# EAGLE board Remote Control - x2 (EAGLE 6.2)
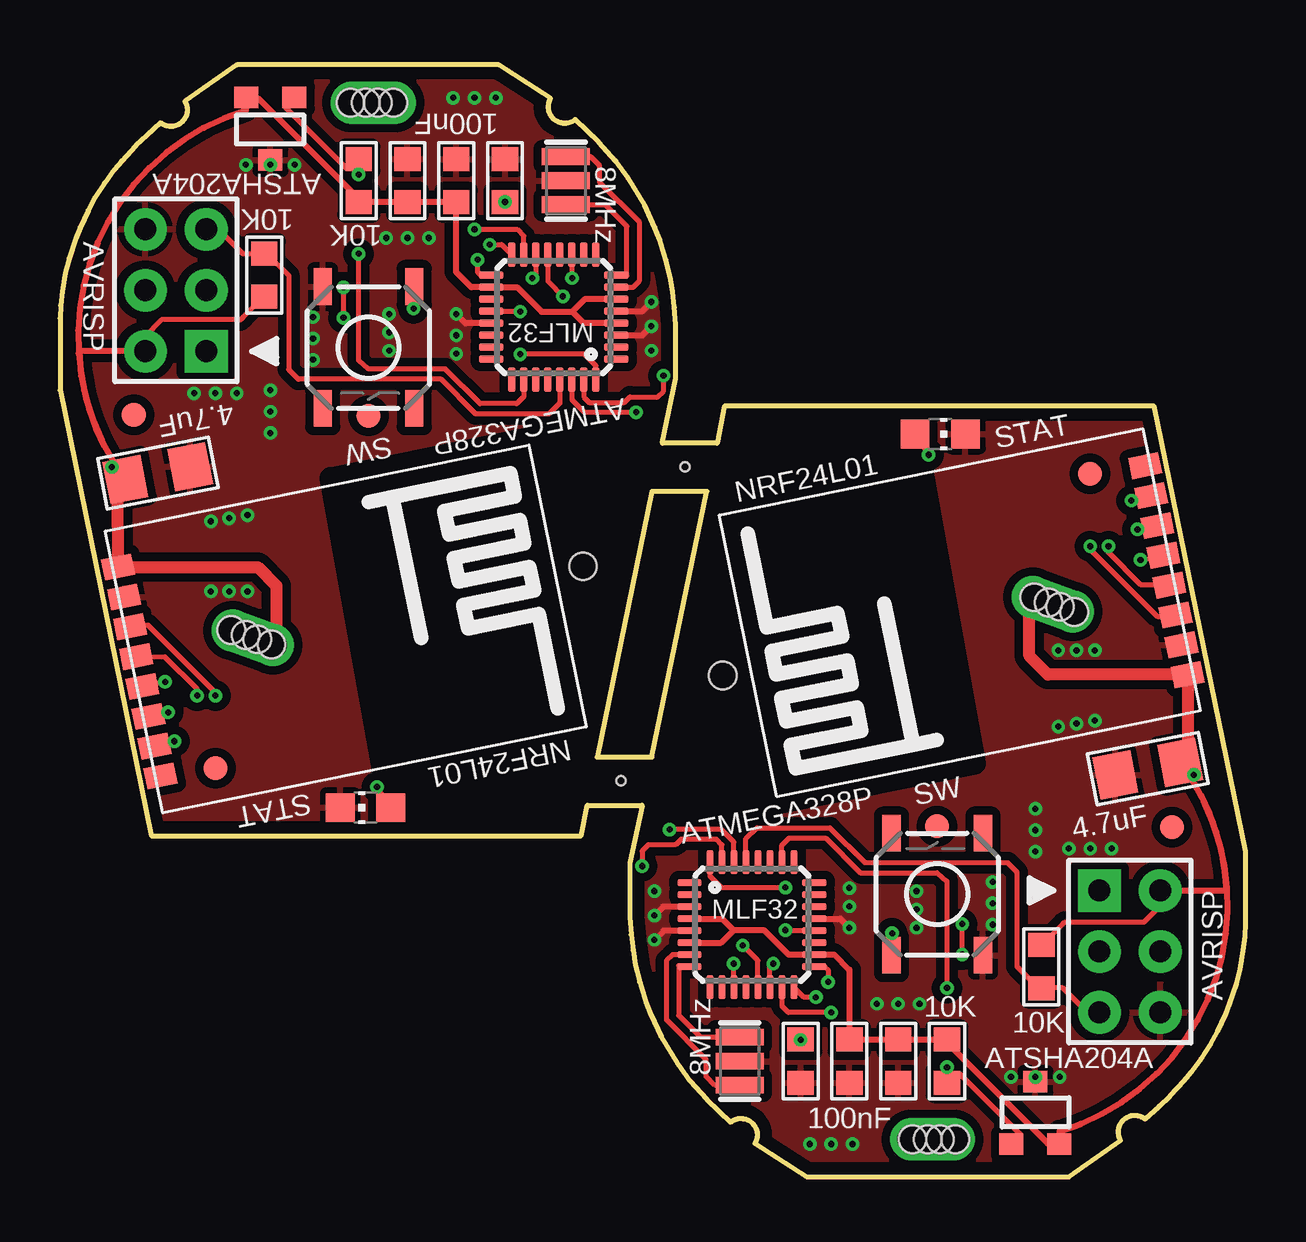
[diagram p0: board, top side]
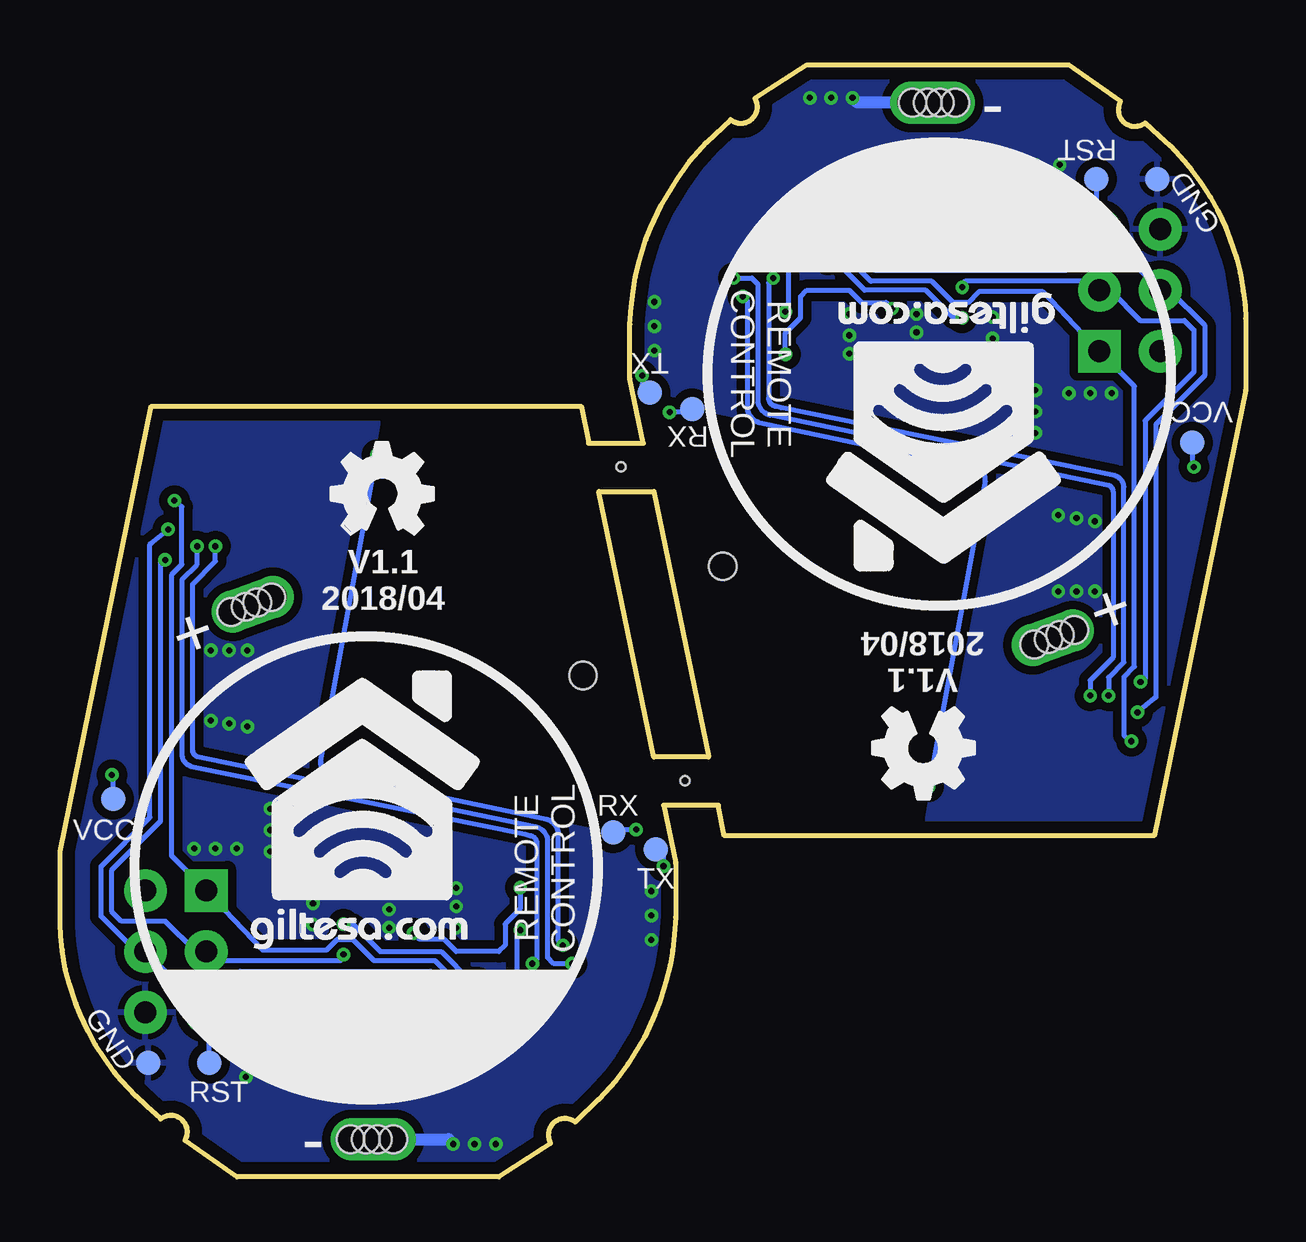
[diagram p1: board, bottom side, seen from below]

Size 49.4 x 46.35 mm. Coordinates in mm from the lower left corner, seen from the top.
Outline: 79 segments
Copper layers (1*16): Top 0.035mm / dielectric 1.6mm / Bottom 0.035mm
Design rules: minimum track width 6mil, minimum drill 12mil, track to track 6mil, track to pad 6mil, pad to pad 6mil, via to via 8mil, smd to smd 0mil, copper to edge 20mil, drill to drill 10mil, minimum pad ring 6mil, minimum via ring 6mil, stop-mask expansion 0mil, vias tented up to drill 100mil, thermal gap 10mil
Net classes: 2 gnd: width 0.305 mm, drill 0.406 mm, clearance 0.203 mm; 3 usbvcc: width 0.203 mm, drill 0.406 mm, clearance 0.203 mm; 4 USBpair: width 0.254 mm, drill 0.406 mm, clearance 0.61 mm
Holes 1.14 mm at 27.61,20.9 21.79,25.45
Holes 0.38 mm at 23.37,16.51 26.04,29.59
tRestrict: 8 lines
bRestrict: 8 lines

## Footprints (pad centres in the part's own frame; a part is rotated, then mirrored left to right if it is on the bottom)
C1206 = smd 1.6 x 1.8: 1 -1.362,0; 2 1.387,0
C0603 = smd 1 x 1.1: 1 -0.901,0; 2 0.901,0
PAD_KEYFINDER = drill 1.143 pad 1.778 offset: P$2 -0.889,0; P$3 0.889,0 | hole 1.143: -0.191,0; 0.318,0; -0.826,0; 0.953,0
HEAD3X2 = drill 0.914 pad 1.778 square: 1 0,0 | drill 0.914 pad 1.778: 2 0,2.54; 3 2.54,0; 4 2.54,2.54; 5 5.08,0; 6 5.08,2.54
CHIP-LED0805 = smd 1.2 x 1.2: A 0,-1.05; C 0,1.05
R0603 = smd 1 x 1.1: 1 -0.901,0; 2 0.901,0
SWITCH-5X5MM-SMD = smd 1.524 x 0.762: A -2.54,1.905; B -2.54,-1.905; NC@1 2.54,1.905; NC@2 2.54,-1.905
PAD.03X.04 = smd 1.016 x 1.016: P$1 0,0
SOT23-3 = smd 1 x 0.9: 1 -1,-1.3; 2 1,-1.3; 3 0,1.3
NRF24L01_SMD = smd 0.9 x 1.27: 3.3V 1.575,0.203; CE 4.115,0.203; CSN 5.385,0.203; GND 2.845,0.203; IRQ 10.465,0.203; MISO 9.195,0.203; MOSI 7.925,0.203; SCK 6.655,0.203
MLF32_HAND_SOLDERING = smd 1.016 x 0.3: 1 -2.604,1.75; 2 -2.604,1.25; 3 -2.604,0.75; 4 -2.604,0.25; 5 -2.604,-0.25; 6 -2.604,-0.75; 7 -2.604,-1.25; 8 -2.604,-1.75; 17 2.604,-1.75; 18 2.604,-1.25; 19 2.604,-0.75; 20 2.604,-0.25; 21 2.604,0.25; 22 2.604,0.75; 23 2.604,1.25; 24 2.604,1.75 | smd 0.3 x 1.016: 9 -1.75,-2.604; 10 -1.25,-2.604; 11 -0.75,-2.604; 12 -0.25,-2.604; 13 0.25,-2.604; 14 0.75,-2.604; 15 1.25,-2.604; 16 1.75,-2.604; 25 1.75,2.604; 26 1.25,2.604; 27 0.75,2.604; 28 0.25,2.604; 29 -0.25,2.604; 30 -0.75,2.604; 31 -1.25,2.604; 32 -1.75,2.604
FIDUCIAL-1X2 = smd 1 x 1: 1 0,0
RESONATOR = smd 0.7 x 2: 1 -1,0; 2 0,0; 3 1,0

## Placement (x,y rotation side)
C1  4.7uF  [C1206]  45.34,17.02 191 top
C2  4.7uF  [C1206]  4.06,29.34 11 top
C3  100nF  [C0603]  30.86,4.83 90 top
C4  100nF  [C0603]  32.89,4.83 90 top
C5  100nF  [C0603]  14.48,41.53 270 top
C6  100nF  [C0603]  18.54,41.53 270 top
C7  100nF  [C0603]  34.92,4.83 90 top
C8  100nF  [C0603]  16.51,41.53 270 top
J1  B-  [PAD_KEYFINDER]  36.35,1.57 0 top
J2  B+  [PAD_KEYFINDER]  41.37,23.88 340 top
J3  B-  [PAD_KEYFINDER]  13.06,44.78 180 top
J4  AVRISP  [HEAD3X2]  43.31,11.94 270 top
J5  B+  [PAD_KEYFINDER]  8.03,22.48 160 top
J6  AVRISP  [HEAD3X2]  6.1,34.42 90 top
L1  STAT  [CHIP-LED0805]  36.68,30.96 270 top
L2  STAT  [CHIP-LED0805]  12.73,15.39 90 top
LOGO1  OSHW_LOGO_FILLX0150-NT  [OSHW_FILLX150_NOTEXT]  38.1,26.8 0 bottom
LOGO2  OSHW_LOGO_FILLX0150-NT  [OSHW_FILLX150_NOTEXT]  11.3,19.56 180 bottom
R1  10K  [R0603]  12.45,41.53 90 top
R2  10K  [R0603]  8.51,37.59 270 top
R3  10K  [R0603]  36.96,4.83 270 top
R4  10K  [R0603]  40.89,8.76 90 top
S1  SW  [SWITCH-5X5MM-SMD]  36.55,11.79 90 top
S2  SW  [SWITCH-5X5MM-SMD]  12.85,34.57 270 top
TP1  RX  [PAD.03X.04]  26.35,14.35 0 bottom
TP2  TX  [PAD.03X.04]  24.57,13.65 0 bottom
TP3  RESET  [PAD.03X.04]  43.18,4.76 0 bottom
TP4  VCC  [PAD.03X.04]  47.18,15.75 0 bottom
TP5  GND  [PAD.03X.04]  45.72,4.76 0 bottom
TP6  RX  [PAD.03X.04]  23.05,32 180 bottom
TP7  TX  [PAD.03X.04]  24.83,32.7 180 bottom
TP8  RESET  [PAD.03X.04]  6.22,41.59 180 bottom
TP9  VCC  [PAD.03X.04]  2.22,30.61 180 bottom
TP10  GND  [PAD.03X.04]  3.68,41.59 180 bottom
U1  ATSHA204A  [SOT23-3]  8.76,43.69 180 top
U2  NRF24L01  [NRF24L01_SMD]  47.5,19.43 101.5 top
U3  ATSHA204A  [SOT23-3]  40.64,2.67 0 top
U4  NRF24L01  [NRF24L01_SMD]  1.91,26.92 281.5 top
U5  ATMEGA328P  [MLF32_HAND_SOLDERING]  28.83,10.52 0 top
U6  ATMEGA328P  [MLF32_HAND_SOLDERING]  20.57,35.84 180 top
U$1  DOMOTICA10MM  [DOMOTICA-10MM]  7.62,36.96 180 bottom
U$2  FIDUCIAL1X2  [FIDUCIAL-1X2]  12.85,31.72 180 top
U$3  FIDUCIAL1X2  [FIDUCIAL-1X2]  6.48,17.04 180 top
U$4  FIDUCIAL1X2  [FIDUCIAL-1X2]  3.07,31.78 180 top
U$5  DOMOTICA10MM  [DOMOTICA-10MM]  41.78,9.4 0 bottom
U$6  FIDUCIAL1X2  [FIDUCIAL-1X2]  36.55,14.63 0 top
U$7  FIDUCIAL1X2  [FIDUCIAL-1X2]  42.93,29.31 0 top
U$8  CC-NC-BCNIX  [CC-NC-B_NIX]  -0.38,0 180 top
U$14  FIDUCIAL1X2  [FIDUCIAL-1X2]  46.33,14.58 0 top
U$15  CC-NC-BCNIX  [CC-NC-B_NIX]  23.75,0 0 top
Y1  8MHz  [RESONATOR]  28.32,4.83 90 top
Y2  8MHz  [RESONATOR]  21.08,41.53 270 top

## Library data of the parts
C1-C8 J1-J3 J5 R1-R4 S1 S2 U2 U4-U6 = ,giltesa
J4 J6 = MyCON2
L1 L2 = led
LOGO1 LOGO2 = ohw-logo
TP1-TP10 = SparkFun-Connectors
U1 U3 = TD-MySensors
U$1 U$5 = ,giltesa_logos
U$2-U$4 U$6 U$7 U$14 = SparkFun
U$8 U$15 = cc-by-nc-sa
Y1 Y2 = MySMD2

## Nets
A3_ATSHA204A: R3.2 U3.1 U5.26
A3_ATSHA204A1: R1.2 U1.1 U6.26
D2_INT_SW: S1.A U5.32
D2_INT_SW1: S2.A U6.32
D7_RF_CE: U2.CE U5.11
D7_RF_CE1: U4.CE U6.11
D9_LEDB~: L1.A U5.13
D9_LEDB~1: L2.A U6.13
D10_RF_CS: U2.CSN U5.14
D10_RF_CS1: U4.CSN U6.14
D11_MOSI: J4.4 U2.MOSI U5.15
D11_MOSI1: J6.4 U4.MOSI U6.15
D12_MISO: J4.1 U2.MISO U5.16
D12_MISO1: J6.1 U4.MISO U6.16
D13_SCK: J4.3 U2.SCK U5.17
D13_SCK1: J6.3 U4.SCK U6.17
GND [gnd]: C1.2 C3.1 C4.1 C7.1 J1.P$2 J4.6 L1.C S1.B TP5.P$1 U2.GND U3.3 U5.3 U5.5 U5.21 Y1.2
GND1 [gnd]: C2.2 C5.1 C6.1 C8.1 J3.P$2 J6.6 L2.C S2.B TP10.P$1 U1.3 U4.GND U6.3 U6.5 U6.21 Y2.2
N$1: TP1.P$1 U5.30
N$2: TP2.P$1 U5.31
N$3: C6.2 U6.20
N$4: TP6.P$1 U6.30
N$5: TP7.P$1 U6.31
N$6: U6.7 Y2.1
N$7: U6.8 Y2.3
N$29: U5.7 Y1.1
N$30: U5.8 Y1.3
N$33: C3.2 U5.20
RESET: J4.5 R4.1 TP3.P$1 U5.29
RESET1: J6.5 R2.1 TP8.P$1 U6.29
VCC: C1.1 C4.2 C7.2 J2.P$2 J4.2 R3.1 R4.2 TP4.P$1 U2.3.3V U3.2 U5.4 U5.6 U5.18
VCC1: C2.1 C5.2 C8.2 J5.P$2 J6.2 R1.1 R2.2 TP9.P$1 U1.2 U4.3.3V U6.4 U6.6 U6.18

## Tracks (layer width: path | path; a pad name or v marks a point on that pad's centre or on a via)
A3_ATSHA204A  (via drill 0.25)
  Top 0.203: U5.26 30.08,13.82 30.38,14.12 31.9,14.12 33.35,12.68 36.55,12.68 36.96,12.32 v36.96,7.87 | U3.1 40.01,1.73 40.01,1.78 37.46,4.32 37.08,4.32 v36.96,4.57 R3.2
  Bottom 0.203: v36.96,7.87 v36.96,4.57
A3_ATSHA204A1  (via drill 0.25)
  Top 0.203: U6.26 19.32,32.53 19.02,32.23 17.5,32.23 16.05,33.68 12.85,33.68 12.45,34.04 v12.45,38.48 | U1.1 9.4,44.62 9.4,44.58 11.94,42.04 12.32,42.04 v12.45,41.78 R1.2
  Bottom 0.203: v12.45,38.48 v12.45,41.78
D2_INT_SW  (via drill 0.25)
  Top 0.203: U5.32 27.08,12.54 27.56,12.06 v30.23,12.06 | S1.A 34.65,10.13 v34.67,10.16
  Bottom 0.203: v34.67,10.16 34.42,9.91 33.4,9.91 32.89,9.4 31.11,9.4 30.86,9.65 30.86,10.54 30.23,11.18 v30.23,12.06
D2_INT_SW1  (via drill 0.25)
  Top 0.203: U6.32 22.32,33.81 21.84,34.29 v19.18,34.29 | S2.A 14.76,36.22 v14.73,36.2
  Bottom 0.203: v14.73,36.2 14.99,36.45 16,36.45 16.51,36.96 18.29,36.96 18.54,36.7 18.54,35.81 19.18,35.18 v19.18,34.29
D7_RF_CE  (via drill 0.25)
  Top 0.203: U5.11 28.08,8.88 v28.07,8.89 | v42.93,26.29 42.93,26.16 45.72,23.37 46.45,23.37 U2.CE
  Bottom 0.203: v28.07,8.89 28.83,8.89 29.08,9.14 29.08,14.03 arc-70 29.59,14.61 43.69,17.53 arc70 43.88,17.78 43.88,24.7 42.93,25.65 v42.93,26.29
D7_RF_CE1  (via drill 0.25)
  Top 0.203: U6.11 21.32,37.48 v21.34,37.47 | v6.48,20.07 6.48,20.19 3.68,22.99 2.95,22.99 U4.CE
  Bottom 0.203: v21.34,37.47 20.57,37.47 20.32,37.21 20.32,32.32 arc-70 19.81,31.75 5.71,28.83 arc70 5.52,28.57 5.52,21.65 6.48,20.7 v6.48,20.07
D9_LEDB~  (via drill 0.25)
  Top 0.203: v36.2,30.1 L1.A | U5.13 29.08,9.02 v28.45,9.65
  Bottom 0.203: v36.2,30.1 38.54,17.34 arc-90 38.16,16.83 29.15,14.92 arc70 28.64,14.29 28.64,9.84 v28.45,9.65
D9_LEDB~1  (via drill 0.25)
  Top 0.203: v13.21,16.26 L2.A | U6.13 20.32,37.33 v20.95,36.7
  Bottom 0.203: v13.21,16.26 10.86,29.02 arc-90 11.24,29.53 20.26,31.43 arc70 20.76,32.07 20.76,36.51 v20.95,36.7
D10_RF_CS  (via drill 0.25)
  Top 0.203: 46.06,24.89 46.06,24.72 | 46.06,24.72 45.85,24.51 | U5.14 29.58,8.75 v29.72,8.89 | v43.69,26.29 43.69,26.02 45.03,24.68 U2.CSN 46.23,24.72 46.06,24.72
  Bottom 0.203: v29.72,8.89 29.53,9.08 29.53,13.91 arc-70 29.78,14.22 30.04,14.29 43.94,17.12 arc70 44.32,17.59 44.32,24.89 43.69,25.53 v43.69,26.29
D10_RF_CS1  (via drill 0.25)
  Top 0.203: 3.35,21.46 3.35,21.63 | 3.35,21.63 3.56,21.84 | U6.14 19.82,37.6 v19.68,37.47 | v5.71,20.07 5.71,20.33 4.37,21.68 U4.CSN 3.17,21.63 3.35,21.63
  Bottom 0.203: v19.68,37.47 19.88,37.27 19.88,32.45 arc-70 19.62,32.13 19.37,32.07 5.46,29.23 arc70 5.08,28.77 5.08,21.46 5.71,20.83 v5.71,20.07
D11_MOSI  (via drill 0.25)
  Top 0.203: 45.85,27.18 45.85,27.11 U2.MOSI v44.9,26.99 | v32.13,6.86 30.35,6.86 30.08,7.13 U5.15
  Bottom 0.203: v44.9,26.99 45.59,26.42 45.66,26.35 45.66,14.99 47.69,12.95 47.69,10.86 46.23,9.4 J4.4 44.58,8.13 42.35,8.13 41.91,8.57 33.97,8.57 32.26,6.86 v32.13,6.86
D11_MOSI1  (via drill 0.25)
  Top 0.203: 3.56,19.18 3.56,19.24 U4.MOSI v4.51,19.37 | v17.27,39.5 19.05,39.5 19.32,39.22 U6.15
  Bottom 0.203: v4.51,19.37 3.81,19.94 3.75,20 3.75,31.37 1.71,33.4 1.71,35.5 3.17,36.96 J6.4 4.83,38.23 7.05,38.23 7.49,37.78 15.43,37.78 17.14,39.5 v17.27,39.5
D12_MISO  (via drill 0.25)
  Top 0.203: v44.64,28.19 U2.MISO | v31.5,7.49 31,7.49 U5.16
  Bottom 0.203: v44.64,28.19 44.32,27.94 44.32,25.53 44.77,25.08 44.77,13.4 J4.1 42.93,11.56 40.96,9.46 38.29,9.46 37.85,9.91 37.21,9.91 36.32,9.02 33.78,9.02 32.26,7.49 v31.5,7.49
D12_MISO1  (via drill 0.25)
  Top 0.203: v4.76,18.16 U4.MISO | v17.91,38.86 18.41,38.86 U6.16
  Bottom 0.203: v4.76,18.16 5.08,18.41 5.08,20.83 4.63,21.27 4.63,32.96 J6.1 6.48,34.8 8.45,36.89 11.11,36.89 11.56,36.45 12.19,36.45 13.08,37.34 15.62,37.34 17.14,38.86 v17.91,38.86
D13_SCK  (via drill 0.25)
  Top 0.203: v45.02,25.72 U2.SCK | v37.59,9.27 v37.59,10.54 | U5.17 31.87,8.77 32,8.64 v32,8.13
  Bottom 0.203: v45.02,25.72 45.21,25.59 45.21,14.83 47.24,12.8 47.24,11.05 46.85,10.65 45.01,10.65 43.75,9.4 J4.3 42.93,9.02 37.72,9.02 37.59,9.14 v37.59,9.27 | v37.59,10.54 37.21,10.54 36.07,9.4 33.53,9.4 32.26,8.13 v32,8.13
D13_SCK1  (via drill 0.25)
  Top 0.203: v4.38,20.64 U4.SCK | v11.81,37.08 v11.81,35.81 | U6.17 17.53,37.59 17.4,37.72 v17.4,38.23
  Bottom 0.203: v4.38,20.64 4.19,20.77 4.19,31.52 2.16,33.55 2.16,35.31 2.55,35.7 4.39,35.7 5.65,36.96 J6.3 6.48,37.34 11.68,37.34 11.81,37.21 v11.81,37.08 | v11.81,35.81 12.19,35.81 13.33,36.96 15.88,36.96 17.14,38.23 v17.4,38.23
GND  (via drill 0.25)
  Top 0.254: U5.21 32.52,10.77 v32.89,10.39 | U5.5 25.15,10.27 v24.77,9.88 | U5.3 25.13,11.27 v24.77,10.9
  Bottom 0.406: 36.28,1.57 J1.P$2 35.4,1.57
  Bottom 0.508: 35.4,1.57 33.22,1.57 v33.02,1.37
  other vias: 31.24,1.37 32.13,1.37 24.77,11.91 38.86,10.52 38.86,11.4 38.86,12.29 43.12,19.02 42.35,18.9 41.59,18.77 41.59,21.95 42.35,21.95 43.12,21.95 32.89,12.04 32.89,11.28 40.64,15.34 40.64,14.45 40.64,13.56 43.81,13.69 42.93,13.69 42.04,13.69 35.69,11.91 35.69,11.15 35.69,10.39 40.64,4.17 39.62,4.17 41.66,4.17 34.92,7.21 34.04,7.21 35.81,7.21
  pour Bottom (isolate 0.356): 49.15,33.02 23.75,33.02 23.75,0 49.15,0
  pour Top (isolate 0.356): 23.75,33.02 49.15,33.02 49.15,0 23.75,0
GND1  (via drill 0.25)
  Top 0.254: U6.21 16.89,35.59 v16.51,35.97 | U6.5 24.25,36.09 v24.64,36.47 | U6.3 24.27,35.09 v24.64,35.46
  Bottom 0.406: 13.12,44.78 J3.P$2 14.01,44.78
  Bottom 0.508: 14.01,44.78 16.18,44.78 v16.38,44.98
  other vias: 18.16,44.98 17.27,44.98 24.64,34.44 10.54,35.84 10.54,34.95 10.54,34.06 6.29,27.33 7.05,27.46 7.81,27.58 7.81,24.41 7.05,24.41 6.29,24.41 16.51,34.32 16.51,35.08 8.76,31.01 8.76,31.9 8.76,32.79 5.59,32.66 6.48,32.66 7.37,32.66 13.72,34.44 13.72,35.2 13.72,35.97 8.76,42.19 9.78,42.19 7.75,42.19 14.48,39.14 15.37,39.14 13.59,39.14
  pour Bottom (isolate 0.356): 0.25,13.34 25.65,13.34 25.65,46.35 0.25,46.35
  pour Top (isolate 0.356): 25.65,13.34 0.25,13.34 0.25,46.35 25.65,46.35
N$1  (via drill 0.25)
  Top 0.203: U5.30 28.08,13.96 27.56,14.48 v25.4,14.48
  Bottom 0.203: TP1.P$1 26.04,14.35 25.91,14.48 v25.4,14.48
N$2  (via drill 0.25)
  Top 0.203: U5.31 27.58,13.85 27.36,14.07 25.88,14.07 25.65,13.84 24.51,13.84 24.26,13.59 v24.26,12.95
  Bottom 0.203: 24.64,13.59 TP2.P$1 24.26,13.34 v24.26,12.95
N$3  (via drill 0.25)
  Top 0.203: C6.2 18.55,40.63 v18.54,40.64 | v19.18,36.07 19.16,36.09 U6.20
  Bottom 0.203: v18.54,40.64 19.3,39.88 19.3,38.1 19.05,37.85 19.05,36.2 v19.18,36.07
N$4  (via drill 0.25)
  Top 0.203: U6.30 21.32,32.4 21.84,31.88 v24,31.88
  Bottom 0.203: TP6.P$1 23.37,32 23.5,31.88 v24,31.88
N$5  (via drill 0.25)
  Top 0.203: U6.31 21.82,32.51 22.05,32.28 23.52,32.28 23.75,32.51 24.89,32.51 25.15,32.77 v25.15,33.4
  Bottom 0.203: 24.77,32.77 TP7.P$1 25.15,33.02 v25.15,33.4
N$6
  Top 0.203: Y2.1 22.11,42.53 22.48,42.16 22.48,41.47 24.13,39.81 24.13,37.34 23.88,37.09 U6.7
N$7
  Top 0.203: Y2.3 20.97,40.51 22.73,40.51 23.62,39.62 23.62,37.55 23.56,37.59 U6.8
N$29
  Top 0.203: Y1.1 27.29,3.83 26.92,4.19 26.92,4.89 25.27,6.54 25.27,9.02 25.52,9.27 U5.7
N$30
  Top 0.203: Y1.3 28.43,5.84 26.67,5.84 25.78,6.73 25.78,8.8 25.85,8.77 U5.8
N$33  (via drill 0.25)
  Top 0.203: C3.2 v30.86,5.71 | v30.23,10.29 30.25,10.27 U5.20
  Bottom 0.203: v30.86,5.71 30.1,6.48 30.1,8.26 30.35,8.51 30.35,10.16 v30.23,10.29
RESET
  Top 0.203: J4.5 42.8,6.86 41.78,7.87 40.78,7.87 R4.1 40.78,7.86 39.88,8.76 39.88,12.7 39.47,13.11 33.53,13.11 32.08,14.55 29.03,14.55 28.58,14.1 U5.29
  Bottom 0.203: TP3.P$1 43.18,6.73 J4.5
RESET1
  Top 0.203: J6.5 6.6,39.5 7.62,38.48 8.62,38.48 R2.1 8.62,38.49 9.53,37.59 9.53,33.66 9.93,33.25 15.88,33.25 17.32,31.8 20.37,31.8 20.82,32.25 U6.29
  Bottom 0.203: TP8.P$1 6.22,39.62 J6.5
VCC  (via drill 0.25)
  Top 0.203: R4.2 41.78,10.54 41.87,10.63 45.17,10.63 45.85,11.3 J4.2 | v47.24,16.76 47.2,16.76 C1.1
  Top 0.254: U3.2 41.66,1.91 arc110 C1.1 arc-35 48.61,11.94 J4.2 | 40.48,24.2 40.51,24.2 J2.P$2 | 33.01,5.73 33.13,5.73 | 33.13,5.73 33.15,5.71 | 28.07,10.29 29.34,10.29 30.36,9.27 U5.18 32.26,9.27 32.89,8.64 32.89,5.84 33.01,5.73 | 28.07,10.29 27.55,9.77 U5.6 | U5.4 27.59,10.77 28.07,10.29 | C4.2 33.01,5.73 | U3.2 41.3,1.37 | U3.2 41.61,1.4 41.15,1.4 37.08,5.46 37.08,5.6 R3.1 | 33.13,5.73 C7.2 R3.1 | 36.97,5.71 R3.1
  Top 0.406: 41.31,23.9 40.48,23.9 40.48,24.2
  Top 0.508: C1.1 arc90 47,17.61 U2.3.3V 41.16,20.94 40.39,21.72 40.39,24.12 40.48,24.2
  Bottom 0.203: TP4.P$1 47.18,16.7 v47.24,16.76
VCC1  (via drill 0.25)
  Top 0.203: R2.2 7.62,35.81 7.53,35.73 4.23,35.73 3.56,35.05 J6.2 | v2.16,29.59 2.2,29.59 C2.1
  Top 0.254: U1.2 7.75,44.45 arc110 C2.1 arc-35 0.79,34.42 J6.2 | 8.93,22.15 8.89,22.15 J5.P$2 | 16.39,40.63 16.27,40.63 | 16.27,40.63 16.26,40.64 | 21.34,36.07 20.07,36.07 19.04,37.09 U6.18 17.14,37.08 16.51,37.72 16.51,40.51 16.39,40.63 | 21.34,36.07 21.86,36.59 U6.6 | U6.4 21.82,35.59 21.34,36.07 | C8.2 16.39,40.63 | U1.2 8.1,44.99 | U1.2 7.79,44.96 8.25,44.96 12.32,40.89 12.32,40.76 R1.1 | 16.27,40.63 C5.2 R1.1 | 12.43,40.64 R1.1
  Top 0.406: 8.09,22.45 8.93,22.45 8.93,22.15
  Top 0.508: C2.1 arc90 2.41,28.74 U4.3.3V 8.24,25.42 9.02,24.64 9.02,22.24 8.93,22.15
  Bottom 0.203: TP9.P$1 2.22,29.65 v2.16,29.59

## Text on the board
tPlace: MLF32 | MLF32
bPlace: - | RST | GND | TX | REMOTE | CONTROL | VCC | RX | V1.1 | + | 2018/04 | + | 2018/04 | V1.1 | RX | VCC | CONTROL | REMOTE | TX | GND | RST | -
Document: The PCB has to be manufactured with 1mm thickness.

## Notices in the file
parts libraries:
SparkFun-Connectors: Licensing: Creative Commons ShareAlike 4.0 International - https://creativecommons.org/licenses/by-sa/4.0
